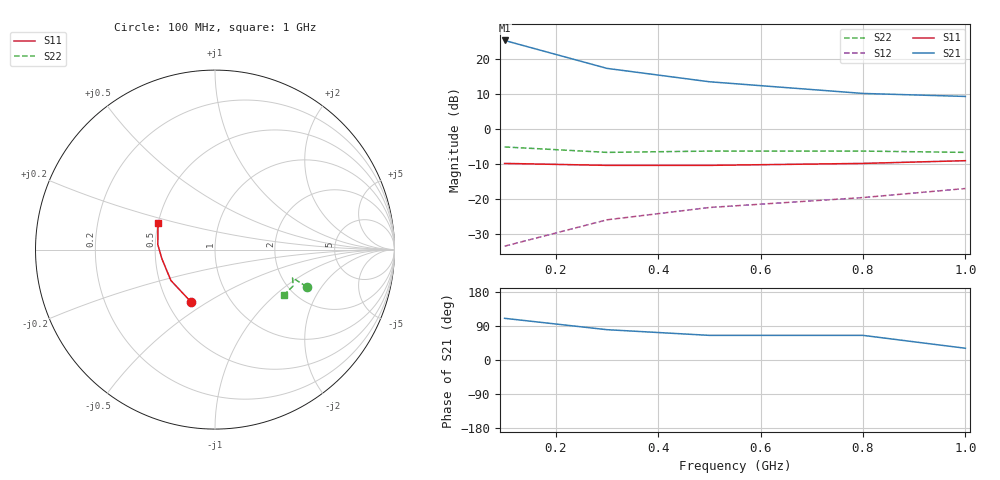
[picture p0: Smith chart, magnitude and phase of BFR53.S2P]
!BFR53
# MHZ S MA R 50
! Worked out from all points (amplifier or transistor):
!   5 points, 100 MHz to 1 GHz, reference 50 ohm
!   highest |S21| = 25.2 dB at 100 MHz (marker M1)
!   |S21| within 3 dB of that: start of sweep to 175.2 MHz
!   unconditionally stable (mu >= 1): 225.7 MHz to 872.9 MHz
!   at 100 MHz: K = 0.87, MSG = 29.4 dB, |S12| = -33.6 dB
!   at 500 MHz: K = 1.04, MAG = 16.7 dB, |S12| = -22.5 dB
!   at 1 GHz: K = 0.91, MSG = 13.2 dB, |S12| = -17.1 dB
100  0.32 -115.0  18.3 110.0  0.021 75.0  0.55 -22.0
300  0.3 -145.0  7.3 80.0  0.05 70.0  0.46 -20.0
500  0.3 -170.0  4.7 65.0  0.075 70.0  0.48 -25.0
800  0.32 175.0  3.2 65.0  0.104 65.0  0.48 -25.0
1000  0.35 155.0  2.9 31.0  0.14 63.0  0.46 -33.0
